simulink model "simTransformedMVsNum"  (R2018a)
settings: Solver=ode15s  StartTime=0.0  StopTime=tsim  MaxStep=1  RelTol=1e-3
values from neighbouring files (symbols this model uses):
  d_step = dnom + dnom.*[0;0]    [runCascade.m]    (also in Main.m = [Fh, Tcin, Thin]; Main_OL.m = [Fh, Tcin+0, Thin]; runTestCalcBlk.m = [Fh, Tcin, Thin])
  dnom = zeros(2,1)    [PI_Tank.m]    (also in runCascade.m)
  Kc = 0    [PI_Tank.m]    (also in runCascade.m = tauQ/(tauC+theta); runTransformedMVs.m = 0.01; Main.m = 1/k*tau/(tauC+theta); runTransf.m = 1/kM(i)*tau(i)/(tauCM(i)+theta(i)))
  p = [V;rho;cp;qnom;MV;transf]    [PI_Tank.m]    (also in runCascade.m = [V;rho;cp;A;tau0;MV;transf]; runTransformedMVs.m = [V;rho;cp;A;tau0;MV;transf]; Main.m = [N, Fc0, rhoc, rhoh,U,A,cpc,cph]; Main_OL.m = [N, Fc0, rhoc, rhoh,U,A,cpc,cph])
  tauI = 1    [PI_Tank.m]    (also in runCascade.m = min(tauQ,4*(tauC+theta)); runTransformedMVs.m = 400; Main.m = min(tau,4*(tauC+theta)); runTransf.m = min(tau(i), 4*(tauCM(i)+theta(i))))
  Tnom = 50    [PI_Tank.m]    (also in runCascade.m; runTransformedMVs.m)
  Tstep = Tnom+10    (= 60)    [PI_Tank.m]    (also in runCascade.m = 40; runTransformedMVs.m = -10)
  tstep_d = 10    [PI_Tank.m]    (also in runCascade.m)
  tstep_T = 50    [PI_Tank.m]    (also in runCascade.m = 500)
  umax = inf    [runCascade.m]    (also in runTransformedMVs.m = 5016)
  vbias = Tnom    (= 50)    [runCascade.m]    (also in runTransformedMVs.m = 0)
undefined symbols (not defined in the file or in its folder): CalcBlock_num, Tank

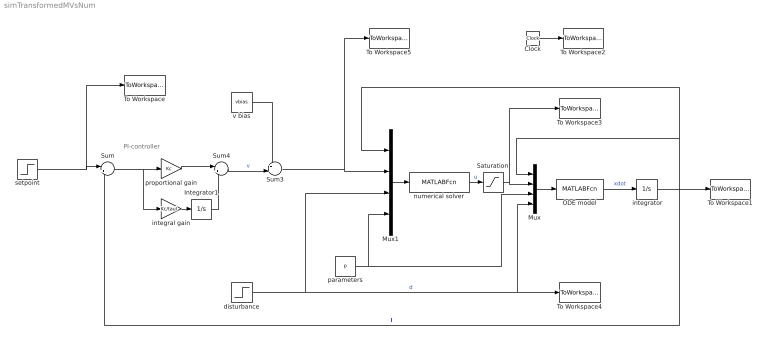
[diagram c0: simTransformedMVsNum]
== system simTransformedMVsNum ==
  note: PI-controller
  " integrator" : Integrator  InitialCondition=Tnom
  Clock : Clock
  Integrator1 : Integrator
  Mux : Mux
  Mux1 : Mux
  ODE model : MATLABFcn  MATLABFcn=Tank(u(1), u(2),u(3:9),u(10:11))  OutputDimensions=1
  Saturation : Saturate  UpperLimit=umax  LowerLimit=0
  Sum : Sum  Inputs=|+-
  Sum3 : Sum  Inputs=++|
  Sum4 : Sum  Inputs=|++
  To Workspace : ToWorkspace  VariableName=Tsp  SampleTime=-1
  To Workspace1 : ToWorkspace  VariableName=T  SampleTime=-1
  To Workspace2 : ToWorkspace  VariableName=time  SampleTime=-1
  To Workspace3 : ToWorkspace  VariableName=u  SampleTime=-1
  To Workspace4 : ToWorkspace  VariableName=d  SampleTime=-1
  To Workspace5 : ToWorkspace  VariableName=v  SampleTime=-1
  disturbance : Step  Time=tstep_d  Before=dnom  After=d_step  SampleTime=0
  integral gain : Gain  Gain=Kc/tauI  Multiplication=Matrix(K*u)
  numerical solver : MATLABFcn  MATLABFcn=CalcBlock_num(u(1),u(2),u(3:4),u(5:11))  OutputDimensions=1
  parameters : Constant  Value=p
  proportional gain : Gain  Gain=Kc  Multiplication=Matrix(K*u)
  setpoint : Step  Time=tstep_T  Before=Tnom  After=Tstep  SampleTime=0
  v bias : Constant  Value=vbias
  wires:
  " integrator"/1 -> Mux/1, Mux1/1, Sum/2, To Workspace1/1  "T"
  Mux/1 -> ODE model/1
  Clock/1 -> To Workspace2/1
  Sum/1 -> integral gain/1, proportional gain/1
  numerical solver/1 -> Saturation/1  "u"
  Sum4/1 -> Sum3/2  "v"
  Mux1/1 -> numerical solver/1
  ODE model/1 -> " integrator"/1  "xdot"
  integral gain/1 -> Integrator1/1
  proportional gain/1 -> Sum4/1
  Integrator1/1 -> Sum4/2
  disturbance/1 -> Mux/4, To Workspace4/1, Mux1/3  "d"
  parameters/1 -> Mux/3, Mux1/4
  v bias/1 -> Sum3/1
  setpoint/1 -> To Workspace/1, Sum/1
  Saturation/1 -> Mux/2, To Workspace3/1
  Sum3/1 -> Mux1/2, To Workspace5/1
